{attribute 'qualified_only'}
{attribute 'strict'}
TYPE eErrorCodesMIS :
(
	ModeChangeEnableFailed := -11,
	ModeChangeFailed := -12,
	ModeChangeDisableFailed := -13,
	ModePosErrWriteAccel := -21,
	ModeHomeHomingFailed := -31,
	ModeHomeErrWritingSpeed := -32,
	ModeHomeErrWritingCrawl := -33,
	ModeHomeErrWritingAccel := -34,
	ModeHomeErrWritingmode  := -35,
	ModeHomeErrWritingPosOffs := -36,
	ModeHomeErrWritingTorque := -37,
	None := 0
);
END_TYPE
